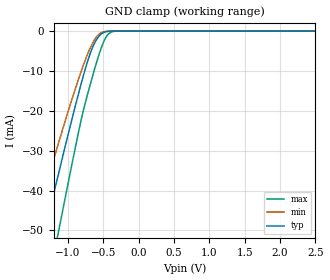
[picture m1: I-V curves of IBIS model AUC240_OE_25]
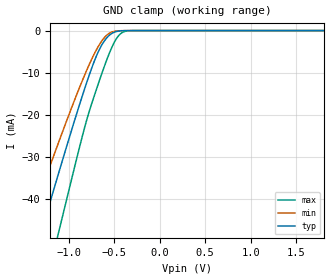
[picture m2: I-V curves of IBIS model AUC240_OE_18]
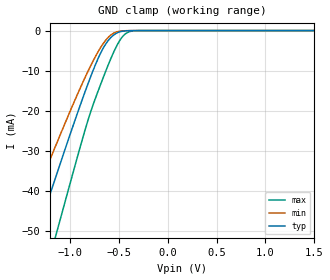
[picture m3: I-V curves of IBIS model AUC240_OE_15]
| TEXAS INSTRUMENTS INCORPORATED
| Standard Linear and Logic Group
| IBIS Model of SN74AUC240
| Octal Buffer/Driver with 3-State Outputs
| This file contains package information for the following:
|  QFN 20-pin (RGY) package as [Component] AUC240_RGY
| This device can be powered at the following Vccs:
|  2.5 volt Vcc
|  1.8 volt Vcc
|  1.5 volt Vcc
|  1.2 volt Vcc
|  0.8 volt Vcc
| This file provides unique models under the [Model Selector] for each Vcc.
| For operation at a specific Vcc, select the appropriate model after each
| [Model Selector] keyword.
[IBIS Ver]   3.2
[Comment char]  |_char
[File Name]   sn74auc240.ibs
[File Rev]   1.1 | x_die
[Date]   March 1, 2003
[Source]   Data created from TI-SPICE simulations at TI-SLL.
[Notes]   The following is an IBIS list for the AUC240.
   Please contact sllibis@ti.com with questions and
   comments concerning SLL IBIS models.
   -The waveforms for the AUC240_OUT Power Clamp ,Pullup, and
   Pulldown are caused by the circuitry that helps reduce
   overshoot and undershoot in transmission lines (EMI).
   These waveforms are norimal for this particular design.
   -Power clamp data deleted as there is no power-clamp diode.
   -End point warning due to AC and DC mismatch.
[Disclaimer] Property of Texas Instruments Incorporated.  Unauthorized
   reproduction and/or distribution is strictly prohibited.
   This product is protected under copyright law.
   Created  2002, (C) Copyright  2002, Texas Instruments
   Incorporated, All Rights Reserved
   UNLESS THERE IS A SIGNED, WRITTEN AGREEMENT TO THE
   CONTRARY, TEXAS INSTRUMENTS (TI) IS PROVIDING THE IBIS
   MODELS  AND WITHOUT ANY WARRANTY, EXPRESSED OR
   IMPLIED.  TI assumes no liability for:
   1) the accuracy of the IBIS models provided to your
   company;
   2) the proper functioning of these IBIS Models in your
   design or for any resulting applications; or
   3) infringement of patents, copyrights or intellectual
   property rights resulting from your use of these IBIS
   models.
   TI provides IBIS Models as a service to our customers.
   You and your company shall not distribute, sell or give
   these models to anyone else without prior written
   permission from TI.
   TI reserves the right to make changes to our products or
   to discontinue any semiconductor product or service
   without notice, and advises our customers to obtain the
   latest version of relevant information to verify, before
   placing orders, that the information being relied on is
   current.
   Please be aware that your receipt and use of the IBIS
   information provided shall serve as acceptance of these
   terms and conditions.  If you do not accept these terms,
   you should return or destroy the IBIS models and any
   other accompanying information immediately.
| Component AUC240_RGY 20-pin QFN
[Component]   AUC240_RGY
[Manufacturer]   Texas Instruments, Inc.
[Package]
|   typ   min   max
R_pkg   0.046   0.035   0.058
L_pkg   1.131nH   0.880nH   1.396nH
C_pkg   0.165pF   0.142pF   0.175pF
[Pin]   signal_name   model_name   R_pin   L_pin   C_pin
1   1NOE   AUC240_OE   0.053   1.289nH   0.142pF
2   1A1   AUC240_IN   0.058   1.386nH   0.172pF
3   2Y4   AUC240_OUT   0.046   1.111nH   0.173pF
4   1A2   AUC240_IN   0.039   0.965nH   0.161pF
5   2Y3   AUC240_OUT   0.035   0.881nH   0.165pF
6   1A3   AUC240_IN   0.035   0.880nH   0.165pF
7   2Y2   AUC240_OUT   0.039   0.961nH   0.161pF
8   1A4   AUC240_IN   0.045   1.105nH   0.172pF
9   2Y1   AUC240_OUT   0.058   1.386nH   0.172pF
10   GND   GND   0.056   1.352nH   0.159pF
11   2A1   AUC240_IN   0.053   1.287nH   0.155pF
12   1Y4   AUC240_OUT   0.058   1.396nH   0.172pF
13   2A2   AUC240_IN   0.047   1.129nH   0.175pF
14   1Y3   AUC240_OUT   0.040   0.976nH   0.164pF
15   2A3   AUC240_IN   0.035   0.884nH   0.169pF
16   1Y2   AUC240_OUT   0.035   0.881nH   0.168pF
17   2A4   AUC240_IN   0.039   0.967nH   0.162pF
18   1Y1   AUC240_OUT   0.046   1.118nH   0.174pF
19   2NOE   AUC240_OE   0.058   1.396nH   0.175pF
20   VCC   POWER   0.052   1.276nH   0.144pF
| Model AUC240_OE
[Model Selector]   AUC240_OE
AUC240_OE_25   2.5 volt Vcc
AUC240_OE_18   1.8 volt Vcc
AUC240_OE_15   1.5 volt Vcc
AUC240_OE_12   1.2 volt Vcc
AUC240_OE_08   0.8 volt Vcc
| Model AUC240_IN
[Model Selector]   AUC240_IN
AUC240_IN_25   2.5 volt Vcc
AUC240_IN_18   1.8 volt Vcc
AUC240_IN_15   1.5 volt Vcc
AUC240_IN_12   1.2 volt Vcc
AUC240_IN_08   0.8 volt Vcc
| Model AUC240_OUT
[Model Selector]   AUC240_OUT
AUC240_OUT_25   2.5 volt Vcc
AUC240_OUT_18   1.8 volt Vcc
AUC240_OUT_15   1.5 volt Vcc
AUC240_OUT_12   1.2 volt Vcc
AUC240_OUT_08   0.8 volt Vcc
| Models and submodels in the file (15): AUC240_OE_25 (Input), AUC240_OE_18 (Input), AUC240_OE_15 (Input), AUC240_OE_12 (Input), AUC240_OE_08 (Input), AUC240_IN_25 (Input), AUC240_IN_18 (Input), AUC240_IN_15 (Input), AUC240_IN_12 (Input), AUC240_IN_08 (Input), AUC240_OUT_25 (3-state), AUC240_OUT_18 (3-state), AUC240_OUT_15 (3-state), AUC240_OUT_12 (3-state), AUC240_OUT_08 (3-state)
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[Model]   AUC240_OE_25
Model_type  Input
Vinl=0.7
Vinh=1.7
| variable   typ   min   max
C_comp   2.39pF   1.91pF   2.79pF
[Temperature Range]   40   100   -40
| Ambient temperature   25   85   -40
[Voltage range]   2.5   2.3   2.7
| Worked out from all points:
|   GND clamp passes 1 mA (typ) near -0.55 V on its own axis
[GND Clamp]
| AUC240_OE_25
|   Voltage   I(typ)   I(min)   I(max)
-3.6V     -222.3mA   -186.1mA   -267.5mA
-1.49V    -62.29mA   -49.79mA   -82.1mA
-1.35V    -51.8mA    -41.14mA   -69.63mA
-1.305V   -48.45mA   -38.39mA   -65.61mA
-1.17V    -38.46mA   -30.25mA   -53.55mA
-1.12V    -34.79mA   -27.28mA   -49.08mA
-735mV    -8.324mA   -6.331mA   -16.67mA
-635mV    -3.426mA   -2.471mA   -10.25mA
-525mV    -682.5uA   -360.4uA   -4.021mA
-430mV    -73.19uA   -34.73uA   -776.9uA
-325mV    -3.339uA   -2.006uA   -30.74uA
2.5V      313.9pA    400.9pA    470.4pA
[Model]   AUC240_OE_18
Model_type  Input
Vinl=0.5775
Vinh=1.2675
| variable   typ   min   max
C_comp   2.44pF   2.00pF   2.80pF
[Temperature Range]   40   100   -40
| Ambient temperature   25   85   -40
[Voltage range]   1.8   1.65   1.95
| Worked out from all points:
|   GND clamp passes 1 mA (typ) near -0.55 V on its own axis
[GND Clamp]
| AUC240_OE_18
|   Voltage   I(typ)   I(min)   I(max)
-3.6V     -222.3mA   -186.1mA   -267.5mA
-1.475V   -61.16mA   -48.85mA   -80.77mA
-1.43V    -57.79mA   -46.07mA   -76.76mA
-1.295V   -47.7mA    -37.79mA   -64.71mA
-1.145V   -36.62mA   -28.76mA   -51.31mA
-1.095V   -32.97mA   -25.81mA   -46.85mA
-830mV    -14.31mA   -10.96mA   -23.64mA
-685mV    -5.607mA   -4.224mA   -13.41mA
-560mV    -1.272mA   -753.7uA   -5.827mA
-485mV    -290.6uA   -140.2uA   -2.305mA
-420mV    -55.81uA   -26.72uA   -608.5uA
1.8V      203.2pA    297.2pA    235.5pA
[Model]   AUC240_OE_15
Model_type  Input
Vinl=0.49
Vinh=1.04
| variable   typ   min   max
C_comp   2.48pF   2.04pF   2.87pF
[Temperature Range]   40   100   -40
| Ambient temperature   25   85   -40
[Voltage range]   1.5   1.4   1.6
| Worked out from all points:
|   GND clamp passes 1 mA (typ) near -0.55 V on its own axis
[GND Clamp]
| AUC240_OE_15
|   Voltage   I(typ)   I(min)   I(max)
-3.6V     -222.3mA   -186.1mA   -267.5mA
-1.505V   -63.42mA   -50.72mA   -83.44mA
-1.325V   -49.94mA   -39.61mA   -67.39mA
-1.17V    -38.46mA   -30.25mA   -53.55mA
-1.12V    -34.79mA   -27.28mA   -49.08mA
-840mV    -14.98mA   -11.48mA   -24.46mA
-695mV    -6.114mA   -4.621mA   -14.06mA
-570mV    -1.487mA   -911.6uA   -6.381mA
-495mV    -364.6uA   -178.8uA   -2.692mA
-430mV    -73.19uA   -34.73uA   -776.9uA
-280mV    -781.4nA   -556.3nA   -5.358uA
1.5V      165.9pA    258.5pA    172.1pA
